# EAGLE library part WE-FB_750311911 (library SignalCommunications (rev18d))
WE-FB Flyback Transformer suitable for LT3573/ LT3574/ LT3575/ LT3748 Characteristics easy design in solution less external components needed small board space low cost no optocoupler needed! long term reliability voltage control no aging same external parts for different output voltages easy design of custom power supply due to standard circuit and change of transformers and two components for feedback loop Isolation voltage up to 2.5 kV Applications Isolated power design Sensor interfaces Isolated telecom converters Power over Ethernet Details see: http://katalog.we-online.de/en/pbs/WE-FB_Linear? Updated 2015-04-03 2015 (C) Wurth Elektronik
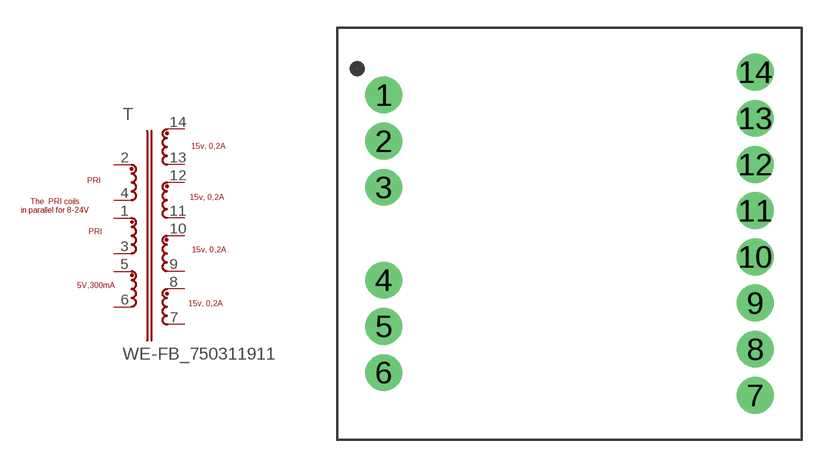
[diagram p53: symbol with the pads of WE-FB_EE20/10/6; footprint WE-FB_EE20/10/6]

Designator prefix T

## WE-FB_750311911_750311911  [WE-FB_EE20/10/6]
1  13  pas
2  1  pas
3  12  pas
4  14  pas
5  11  pas
6  10  pas
7  9  pas
8  8  pas
9  7  pas
10  6  pas
11  5  pas
12  4  pas
13  3  pas
14  2  pas

## Footprint WE-FB_EE20/10/6 (pad centres in mm)
drill 1.32: 1 -10,7.48; 2 -10,4.99; 3 -10,2.5; 4 -10,-2.5; 5 -10,-4.99; 6 -10,-7.48; 7 10,-8.715; 8 10,-6.225; 9 10,-3.735; 10 10,-1.245; 11 10,1.245; 12 10,3.735; 13 10,6.225; 14 10,8.715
